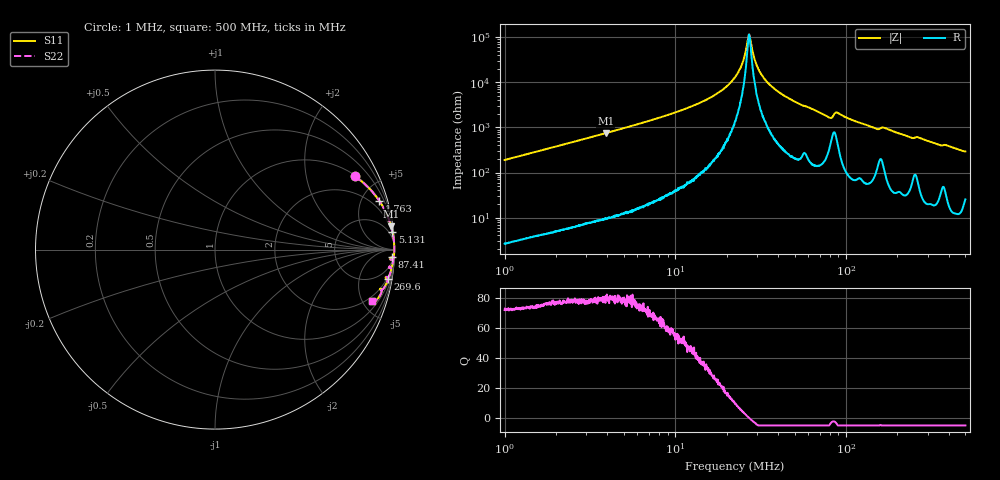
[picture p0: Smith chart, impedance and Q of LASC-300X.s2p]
!s-Parameter Generated by FASTRON Sdn. Bhd.
!FASTRON P/N : LASC-300X
!Keysight Technologies,E4991B,MY54100416,A.01.15
!Date: Tue Mar 17 14:18:27 2026
!Version  : Rev00 Tue Mar 17 14:18:27 2026
!Data & Calibration Information:
!PortZ  Port1:50+j0  Port2:50+j0
!When reading, reference impedance value at option line is always used.
! Remarks : This data is being provided solely for informational purposes.
!Freq	S11	S21	S12	S22
# Hz S dB R 50
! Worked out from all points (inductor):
!   1601 points, 1 MHz to 500 MHz, reference 50 ohm
!   read as one part in series: L = 30.1 uH near 1.032 MHz
!   highest Q = 81 at 3.909 MHz (marker M1), where L = 30.5 uH
!   self-resonance near 27.05 MHz
!   S11 on the Smith chart (normalised r, x): 1 MHz: 1.05, +3.79; 1.763 MHz: 1.09, +6.67; 5.131 MHz: 1, +20; 87.41 MHz: 13, -41; 269.6 MHz: 2, -12; 500 MHz: 1.51, -5.87
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1000000  -1.11 27.6  -6.68 -61.6  -6.68 -61.6  -1.11 27.6
1763117  -0.40 16.6  -10.87 -72.6  -10.87 -72.6  -0.40 16.6
2820919  -0.17 10.6  -14.74 -78.7  -14.74 -78.7  -0.17 10.6
3909188  -0.09 7.6  -17.58 -81.7  -17.58 -81.7  -0.09 7.6
5130580  -0.05 5.7  -20.02 -83.5  -20.02 -83.5  -0.05 5.7
7957584  -0.02 3.5  -24.25 -85.6  -24.25 -85.6  -0.02 3.5
1.570294e7  -0.01 1.3  -32.91 -86.9  -32.91 -86.9  -0.01 1.3
1.929232e7  -0.01 0.8  -37.28 -86.2  -37.28 -86.2  -0.01 0.8
2.236068e7  -0.01 0.4  -42.29 -83.5  -42.29 -83.5  -0.01 0.4
2.454537e7  -0.01 0.2  -48.01 -77.8  -48.01 -77.8  -0.01 0.2
2.652813e7  -0.01 0.0  -58.54 -43.1  -58.54 -43.1  -0.01 0.0
2.715362e7  -0.01 -0.0  -60.98 7.3  -60.98 7.3  -0.01 -0.0
3.02733e7  -0.01 -0.3  -46.82 77.8  -46.82 77.8  -0.01 -0.3
3.468165e7  -0.01 -0.6  -40.01 83.8  -40.01 83.8  -0.01 -0.6
4.412501e7  -0.01 -1.2  -33.82 85.5  -33.82 85.5  -0.01 -1.2
6.307767e7  -0.03 -2.2  -28.30 84.5  -28.30 84.5  -0.03 -2.2
7.994179e7  -0.12 -3.3  -24.48 74.5  -24.48 74.5  -0.12 -3.3
8.74121e7  -0.12 -2.5  -26.77 70.7  -26.77 70.7  -0.12 -2.5
1.482463e8  -0.13 -5.9  -19.71 78.7  -19.71 78.7  -0.13 -5.9
1.77937e8  -0.11 -6.3  -19.14 80.4  -19.14 80.4  -0.11 -6.3
2.696248e8  -0.22 -9.5  -15.62 76.5  -15.62 76.5  -0.22 -9.5
5e8  -0.70 -18.2  -10.08 66.9  -10.08 66.9  -0.70 -18.2
